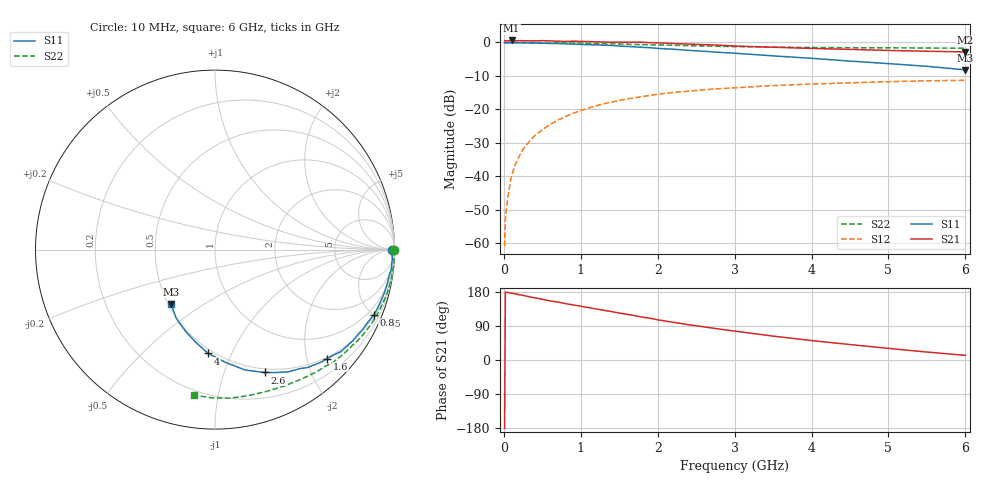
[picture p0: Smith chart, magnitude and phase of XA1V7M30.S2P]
! SIEMENS Discrete & RF Semiconductors
! BFY180
! Si NPN RF Bipolar Junction Transistor in MICRO-X
! VCE = 1.75 V  IC = 0.3 mA
! Common Emitter S-Parameters:  May  1997
# GHz  S  MA  R  50
!  f  S11  S21  S12  S22
! GHz  MAG  ANG  MAG  ANG  MAG  ANG  MAG  ANG
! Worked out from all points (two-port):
!   36 points, 10 MHz to 6 GHz, reference 50 ohm
!   highest |S21| = 0.60 dB at 100 MHz (marker M1); lowest = -2.8 dB at 6 GHz (marker M2)
!   |S21| within 3 dB of the highest: start of sweep to 5.025 GHz
!   lowest |S11| = -8.2 dB at 6 GHz (marker M3), VSWR 2.28, Z = 25.8 - j18.5 ohm
!   |S11| at or under -10 dB: nowhere
!   |S22| runs from -1.7 to 0.0 dB; largest |S21 - S12| = 1.1
!   S11 on the Smith chart (normalised r, x): 10 MHz: open; 800 MHz: 0.58, -4.96; 1.6 GHz: 0.47, -2.39; 2.6 GHz: 0.46, -1.38; 4 GHz: 0.47, -0.82; 6 GHz: 0.52, -0.37
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0.01  0.9882 0.0  1.056 -180.0  0.0009 79.8  0.999 -0.1
0.02  0.9817 -0.3  1.061 179.3  0.0023 90.8  0.9999 -0.5
0.05  0.9866 -1.3  1.057 178.2  0.0048 89.0  1 -1.0
0.1  0.989 -3.0  1.072 176.5  0.0102 90.7  0.997 -2.2
0.15  0.9881 -4.4  1.057 174.5  0.0151 87.4  0.9999 -3.2
0.25  0.9856 -7.4  1.063 170.5  0.0252 84.5  0.9999 -5.4
0.4  0.9784 -11.2  1.057 164.3  0.0403 80.9  0.9963 -8.4
0.6  0.9677 -17.1  1.056 155.9  0.0594 76.0  0.9902 -12.8
0.8  0.9562 -22.5  1.035 148.8  0.0781 71.3  0.9837 -16.9
0.9  0.9437 -25.2  1.045 145.4  0.0873 68.9  0.9792 -19.0
1.1  0.9266 -30.6  1.032 138.2  0.1044 64.1  0.9701 -23.1
1.4  0.9025 -39.1  1.009 127.8  0.1282 57.4  0.953 -29.2
1.6  0.8726 -44.1  1.007 120.6  0.1427 53.5  0.9414 -32.9
1.8  0.8451 -49.7  1.008 113.2  0.1557 49.7  0.9286 -36.5
2.2  0.7937 -59.1  0.966 99.6  0.1791 41.9  0.9096 -43.7
2.6  0.7387 -67.9  0.928 87.4  0.1963 35.4  0.8859 -50.0
3  0.6914 -76.0  0.885 76.3  0.2101 29.2  0.8676 -56.1
3.5  0.6302 -84.8  0.849 63.0  0.2265 22.9  0.8527 -63.0
4  0.58 -93.7  0.815 51.3  0.2389 16.7  0.8408 -69.9
4.5  0.5265 -101.9  0.788 40.8  0.2492 11.0  0.8347 -76.9
5.5  0.4397 -119.4  0.739 21.0  0.2668 0.3  0.8266 -91.1
6  0.3897 -128.9  0.723 12.2  0.272 -5.1  0.8182 -98.2
